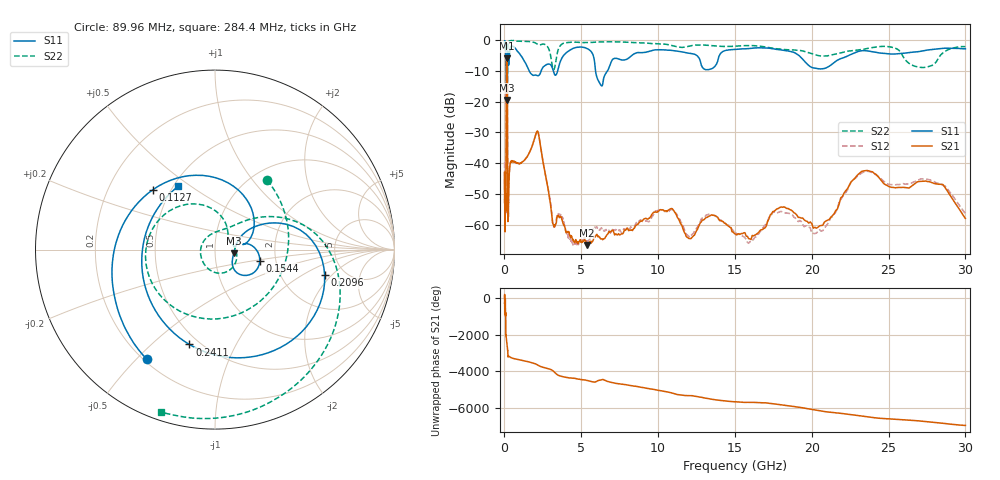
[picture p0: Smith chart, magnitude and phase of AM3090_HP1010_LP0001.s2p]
! Date/Time: Thu, Feb 28, 2019 2:04 PM
! Network Analyzer: Agilent Technologies E8364B Rev: A.07.50.67
! Sweep from 0.010 to 30.000 GHz, 1601 Points, Sweep Type: LOG
! Power Supply: 5.023 V, 0.002 A
# Hz S DB R 50
!freq MagS11 AngS11 MagS21 AngS21 MagS12 AngS12 MagS22 AngS22
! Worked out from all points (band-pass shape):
!   1601 points, 10 MHz to 30 GHz, reference 50 ohm
!   highest |S21| = -5.94 dB at 148.4 MHz (marker M1); lowest = -66.5 dB at 5.365 GHz (marker M2)
!   |S21| within 3 dB of the highest: 125.8 MHz to 181.1 MHz (55.3 MHz wide, 36 % of centre)
!   lowest |S11| = -19.5 dB at 182.2 MHz (marker M3), VSWR 1.24, Z = 61.6 - j2.63 ohm
!   |S11| at or under -10 dB: 1.61 GHz to 2.387 GHz (777.5 MHz wide, 38.9 % of centre); 3.183 GHz to 3.465 GHz (281.2 MHz wide, 8.46 % of centre); 5.927 GHz to 6.709 GHz (781.3 MHz wide, 12.4 % of centre)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
!   |S22| runs from -22.1 to -0.1 dB; largest |S21 - S12| = 0.012
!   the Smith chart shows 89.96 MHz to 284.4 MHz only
!   S11 on the Smith chart (normalised r, x): 89.96 MHz: 0.21, -0.54; 112.7 MHz: 0.40, +0.35; 154.4 MHz: 1.65, -0.22; 209.6 MHz: 3.54, -1.65; 241.1 MHz: 0.44, -0.67; 284.4 MHz: 0.53, +0.45
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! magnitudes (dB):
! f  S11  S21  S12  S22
! 10 MHz  -0.3  -48.3  -39.7  -0.5
! 38.04 MHz  -0.5  -59.3  -61.3  -1.3
! 48.37 MHz  -0.7  -49.0  -48.6  -1.5
! 89.96 MHz  -2.9  -52.1  -52.2  -6.3
! 112.7 MHz  -6.4  -21.5  -21.6  -8.0
! 144.7 MHz  -13.7  -6.0  -5.9  -18.8
! 148.4 MHz  -12.7  -5.9  -5.9  -17.8
! 154.4 MHz  -11.8  -6.0  -6.0  -17.1
! 182.2 MHz  -19.5  -9.3  -9.3  -17.9
! 209.6 MHz  -4.1  -48.6  -48.4  -2.5
! 222.5 MHz  -3.6  -58.2  -57.2  -1.4
! 241.1 MHz  -5.2  -56.9  -55.9  -0.7
! 284.4 MHz  -7.8  -47.4  -47.1  -0.4
! 550.5 MHz  -2.1  -39.5  -39.2  -0.2
! 2.084 GHz  -11.4  -29.9  -29.9  -1.2
! 3.204 GHz  -10.3  -60.1  -60.6  -9.6
! 5.365 GHz  -2.7  -66.5  -65.2  -0.8
! 6.234 GHz  -14.3  -64.4  -61.6  -0.6
! 7.926 GHz  -6.3  -61.5  -61.4  -0.7
! 20.31 GHz  -9.2  -61.0  -62.6  -4.9
! 23.48 GHz  -3.5  -42.4  -42.7  -2.9
! 30 GHz  -2.9  -57.9  -56.4  -2.1
